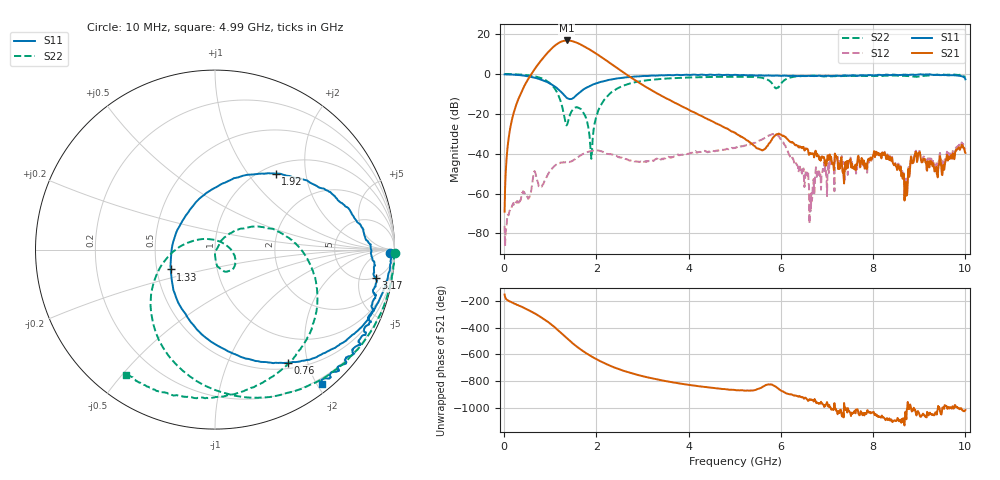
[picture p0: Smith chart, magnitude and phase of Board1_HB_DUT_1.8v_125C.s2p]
! Created Tue May 27 14:50:37 2025
# hz S ma R 50
! 2 Port Network Data from SP1.SP block
! freq  magS11  angS11  magS21  angS21  magS12  angS12  magS22  angS22
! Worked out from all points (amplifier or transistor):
!   1000 points, 10 MHz to 10 GHz, reference 50 ohm
!   highest |S21| = 16.9 dB at 1.36 GHz (marker M1)
!   |S21| within 3 dB of that: 1.079 GHz to 1.739 GHz (659.9 MHz wide, 46.8 % of centre)
!   unconditionally stable (mu >= 1): 15.86 MHz to 47.22 MHz; 51.53 MHz to end of sweep
!   at 1.67 GHz: K = 8.45, MAG = 15.4 dB, |S12| = -40.6 dB
!   at 5.01 GHz: K = 23.08, MAG = -13.0 dB, |S12| = -37.0 dB
!   at 10 GHz: K = 499.74, MAG = -30.9 dB, |S12| = -37.8 dB
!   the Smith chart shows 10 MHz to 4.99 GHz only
!   S11 on the Smith chart (normalised r, x): 10 MHz: 52, -43; 760 MHz: 0.58, -1.68; 1.33 GHz: 0.59, -0.14; 1.92 GHz: 1.14, +1.37; 3.17 GHz: 5, -9; 4.99 GHz: 0.12, -2.07
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1e7  0.9773 -1.1  0.0003514 -151.1  0.0001545 84.6  1.004 -0.9
2e8  0.9644 -13.9  0.09917 145.7  0.0005797 83.6  0.9922 -18.4
5.3e8  0.8721 -37.6  0.7715 92.1  0.0007526 96.0  0.9301 -52.4
7.6e8  0.75 -57.2  1.913 48.0  0.001462 72.9  0.8214 -82.3
9.3e8  0.6308 -74.3  3.315 9.0  0.002748 115.2  0.6655 -110.3
1.09e9  0.4949 -95.7  5.05 -34.1  0.004943 101.4  0.442 -143.8
1.23e9  0.3604 -124.5  6.447 -77.3  0.006023 83.3  0.1989 175.7
1.33e9  0.2701 -155.9  6.936 -109.2  0.006109 76.0  0.05919 107.2
1.36e9  0.251 -168.3  6.971 -118.6  0.00605 75.2  0.05238 58.7
1.51e9  0.2552 125.9  6.527 -163.5  0.007009 75.8  0.1351 -33.8
1.68e9  0.3772 81.5  5.365 152.3  0.009482 66.8  0.1251 -69.1
1.92e9  0.5426 51.4  3.705 100.1  0.01185 41.9  0.02405 43.6
2.26e9  0.7108 27.3  2.021 41.2  0.009838 12.0  0.2961 25.0
2.61e9  0.8211 9.7  1.051 -4.7  0.007646 0.5  0.5233 -6.8
3.17e9  0.9107 -10.1  0.4083 -55.9  0.006576 15.9  0.7138 -44.1
3.34e9  0.9216 -15.6  0.3151 -68.5  0.006956 9.8  0.7454 -53.9
4.99e9  0.9546 -51.5  0.03425 -145.6  0.0141 -13.0  0.8549 -125.3
5.01e9  0.9582 -51.9  0.03294 -147.1  0.01411 -12.1  0.8538 -126.1
5.91e9  0.9188 -70.9  0.03086 -127.9  0.03013 -99.9  0.4462 -146.9
6.67e9  0.8963 -92.2  0.009913 141.4  0.000645 125.0  0.9077 -157.9
8.34e9  0.9417 -134.2  0.007083 -8.7  0.007362 -13.9  0.9134 166.7
1e10  0.7383 -161.5  0.01047 64.1  0.01281 62.0  0.84 151.8
